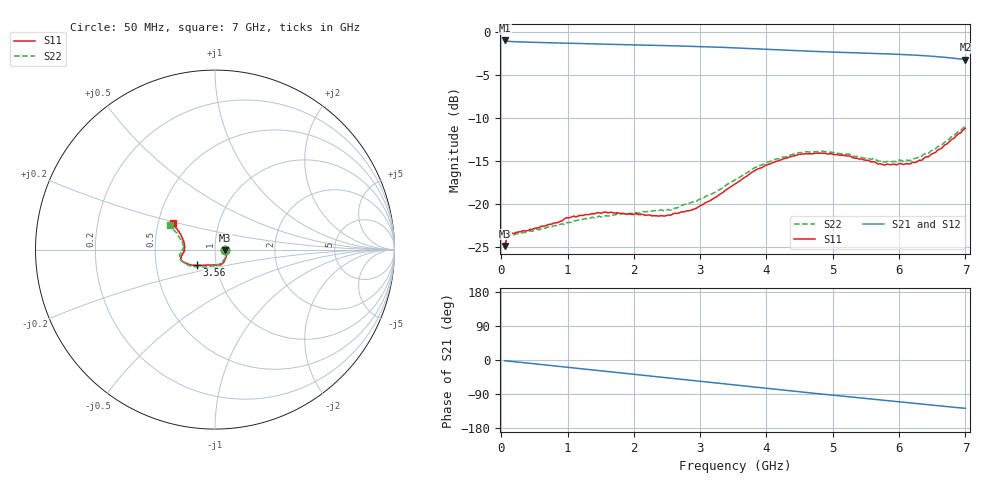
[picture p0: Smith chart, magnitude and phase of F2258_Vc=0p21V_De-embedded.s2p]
! Integrated Device Technology
! Corporate Headquarters
! 6024 Silver Creek Valley Road
! San Jose, CA 95138  USA
! Phone:  1-408-284-8200
! Toll Free:  1-800-223-1366
! Webpage:  http://www.idt.com/
! Timing and RF Division
! 515 Groton Road, Suite 102
! Westford, MA 01886-6024
! Device:  F2258
! Description: Voltage Variable RF Attenuator
! Frequency:  50.0 -  6000.00 MHz
! Package:  3x3 mm Thin QFN Plastic Package: 16 pin
! Ports:  2 RF, 2 DC
!  Pin  1  = NC
!  Pin  2  = NC
!  Pin  3  = RF2  = Port 2
!  Pin  4  = GND
!  Pin  5  = Vdd
!  Pin  6  = NC
!  Pin  7  = VCTRL
!  Pin  8  = NC
!  Pin  9  = GND
!  Pin 10  = RF1  = Port 1
!  Pin 11  = NC
!  Pin 12  = NC
!  Pin 13  = NC
!  Pin 14  = NC
!  Pin 15  = NC
!  Pin 16  = NC
! Vcntrl:  0.210 Volts
! Vdd:  +3.300 Volts
! Current:  1.080 mA
! Data:  The device was measured on a the F2258 evaluation board which has
!  individual transmission lines to the RF pins.  Data was collected
!  using a calibrated network analyzer.  The evaluation board was
!  de-embedded using a TRL calibration technique.
!  The reference plane is the edge of the package pin.
! Misc:  SN 10
!  Action Tracker AT0285
! Date Measured:  2014-12-10
! Date:  2016-01-13  MJV
! Note:
!  Integrated Device Technology supplies this data as a sample of measured
!  data at the package pin for this product.  Your particular data for this
!  product may vary.
!  Data was taken at 25 degrees C.
!  Integrated Device Technology reserves the right to change this data at anytime.
!Freq_(GHz)  S11M_(dB)  S11P_(deg)  S21M_(dB)  S21P_(deg)  S12M_(dB)  S12P_(deg)  S22M_(dB)  S22P_(deg)
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# GHz S dB R 50
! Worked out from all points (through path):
!   201 points, 50 MHz to 7 GHz, reference 50 ohm
!   highest |S21| = -0.96 dB at 50 MHz (marker M1); lowest = -3.2 dB at 7 GHz (marker M2)
!   group delay of S21, straight-line fit = 50.5 ps
!   lowest |S11| = -24.9 dB at 50 MHz (marker M3), VSWR 1.12, Z = 56 - j0.393 ohm
!   |S11| at or under -10 dB: start of sweep to end of sweep
!   |S22| runs from -24.9 to -10.9 dB; largest |S21 - S12| = 0.0004
!   S11 on the Smith chart (normalised r, x): 50 MHz: 1.12, -0.01; 3.56 GHz: 0.81, -0.14; 7 GHz: 0.60, +0.19
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0.05  -24.88 -3.5  -0.96 -1.9  -0.96 -1.9  -24.92 -3.0
0.08475  -23.91 -5.9  -1.03 -2.4  -1.03 -2.4  -23.97 -5.4
0.15425  -23.41 -9.3  -1.08 -3.6  -1.08 -3.6  -23.59 -9.4
0.71025  -22.38 -37.2  -1.22 -14.1  -1.22 -14.1  -22.68 -38.6
0.98825  -21.60 -51.0  -1.27 -19.3  -1.27 -19.3  -22.17 -54.7
1.2315  -21.35 -59.3  -1.32 -23.8  -1.32 -23.8  -21.80 -63.7
1.6485  -20.95 -71.0  -1.41 -31.4  -1.41 -31.4  -21.31 -76.7
2.37825  -21.42 -92.5  -1.54 -44.8  -1.54 -44.8  -20.78 -94.3
2.552  -21.31 -98.4  -1.57 -48.0  -1.57 -48.0  -20.74 -99.6
2.93425  -20.53 -115.1  -1.65 -55.1  -1.65 -55.1  -19.73 -113.0
3.525  -17.69 -137.8  -1.82 -66.2  -1.82 -66.2  -17.21 -135.6
3.55975  -17.50 -138.8  -1.83 -66.9  -1.83 -66.9  -17.03 -136.6
4.0115  -15.43 -151.4  -2.00 -75.2  -2.00 -75.2  -15.12 -151.0
4.46325  -14.28 -159.8  -2.16 -83.4  -2.16 -83.4  -14.07 -162.1
4.7065  -14.14 -163.0  -2.23 -87.7  -2.23 -87.7  -13.96 -166.3
5.2625  -14.42 -170.0  -2.38 -97.4  -2.38 -97.4  -14.21 -174.3
5.6795  -15.35 -176.8  -2.46 -104.6  -2.47 -104.6  -15.03 -179.7
5.85325  -15.41 179.0  -2.52 -107.8  -2.52 -107.8  -15.06 175.7
6.166  -15.34 171.2  -2.63 -113.4  -2.63 -113.4  -14.97 169.8
6.33975  -14.93 164.9  -2.71 -116.5  -2.71 -116.5  -14.43 165.4
6.722  -13.01 153.3  -2.94 -123.1  -2.94 -123.1  -12.71 156.4
7  -11.20 147.9  -3.19 -127.4  -3.19 -127.4  -10.92 151.4
